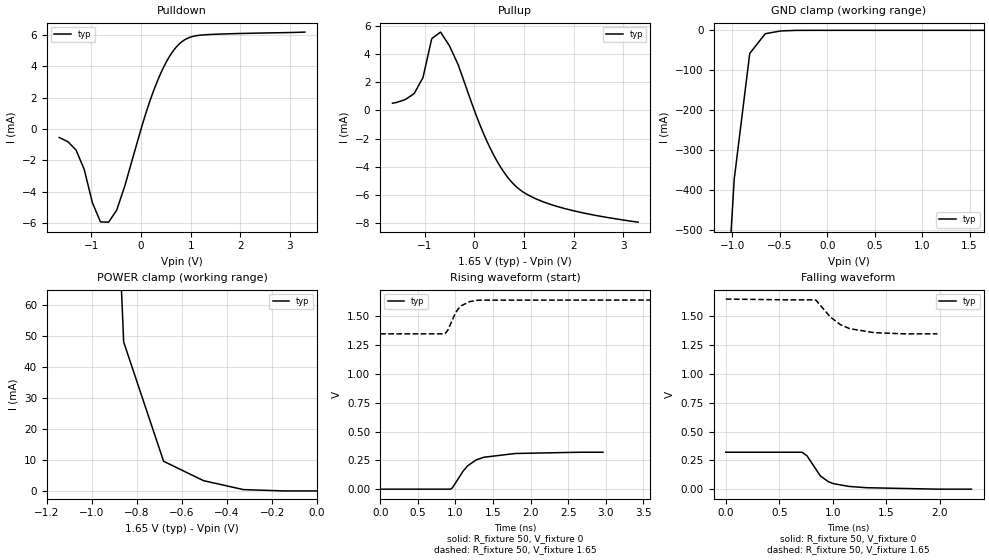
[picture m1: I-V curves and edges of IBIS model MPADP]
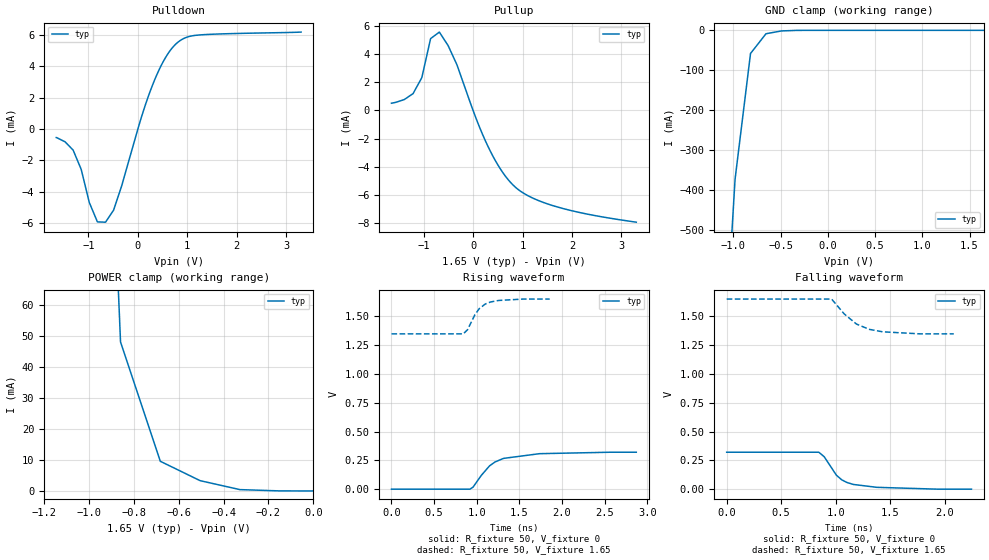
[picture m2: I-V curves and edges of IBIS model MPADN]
| Created by SiliconSmart 2008.10 (Production)
| There are several IBIS sections which it is inappropriate for this tool to
| automatically fill in - copyrights and packaging details are two examples.
| We are making it easy for you to add these things by providing commented-out
| section headers and brief descriptions of each such section.  Of course, the
| IBIS standard is the ultimate section description; these are merely summaries.
[IBIS Ver]   4.1
[File Name]   ss_1p08_1p65_125c.ibs
[File Rev]   1.0
[Date]   December 18 11:21:58
[Source]   From SiliconSmart 2008.10 (Production)
|[Notes]   Use this section for any special notes related to the file.
|   (fill in and uncomment to use this section)
|[Disclaimer]   Legal disclaimer section.
|   (fill in and uncomment to use this section)
|[Copyright]   Copyright 1995, XYZ Corp., All Rights Reserved
|   (fill in and uncomment to use this section)
[Component]   pdqs_ddr2_cl_driver_6p9ma
[Manufacturer]   Unknown
[Package]
| Variable   typ   min   max
R_pkg   18   NA   NA
L_pkg   1n   NA   NA
C_pkg   15f   NA   NA
[Pin]   signal_name   model_name   R_pin   L_pin   C_pin
1   PADP   MPADP   NA   NA   NA
2   PADN   MPADN   NA   NA   NA
3   DVSS   GND   NA   NA   NA
4   DVDD   POWER   NA   NA   NA
|[Package Model]   Package model name.  40-char limit.
|   (fill in and uncomment to use this section)
[Pin Mapping]  pulldown_ref   pullup_ref   gnd_clamp_ref  power_clamp_ref
1   DVSS   DVDD   DVSS   DVDD
2   DVSS   DVDD   DVSS   DVDD
3   DVSS   NC   NC   NC
4   NC   DVDD   NC   NC
[Diff Pin]  inv_pin  vdiff  tdelay_typ tdelay_min tdelay_max
1   2   NA   -36.38p   NA   NA
| Models and submodels in the file (2): MPADP (I/O), MPADN (I/O)
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|PADP pin
[Model]   MPADP
Model_type I/O
Polarity Non-Inverting
Vinl = 0.8
Vinh = 2.0
Vmeas = 0.9
| Capacitance   typ   min   max
C_comp   6.42p   NA   NA
| Variables   typ   min   max
[Temperature Range]   125   NA   NA
[Voltage Range]   1.65   NA   NA
[Pullup Reference]   1.65   NA   NA
[Pulldown Reference]   0.0   NA   NA
[POWER Clamp Reference]   1.65   NA   NA
[GND Clamp Reference]   0.0   NA   NA
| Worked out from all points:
|   slope of the pulldown table from 0 to 0.247 V, typ, clamps not added: 103 ohm
|   slope of the pullup table from 0 to 0.247 V, typ, clamps not added: 115 ohm
|   GND clamp passes 1 mA (typ) near -0.43 V on its own axis
|   POWER clamp passes 1 mA (typ) near -0.36 V on its own axis
|   falling waveform, R_fixture 50, V_fixture 0: 20-80 % time 178ps typ, NA min, NA max; typ from 0.321 V to 0 V
|   falling waveform, R_fixture 50, V_fixture 1.65: 20-80 % time 230ps typ, NA min, NA max; typ from 1.65 V to 1.35 V
|   rising waveform, R_fixture 50, V_fixture 0: 20-80 % time 277ps typ, NA min, NA max; typ from 0 V to 0.321 V
|   rising waveform, R_fixture 50, V_fixture 1.65: 20-80 % time 156ps typ, NA min, NA max; typ from 1.35 V to 1.65 V
[Pulldown]
| Voltage   I(typ)   I(min)   I(max)
-1.65V    -547uA     NA         NA
-1.309V   -1.35mA    NA         NA
-1.145V   -2.589mA   NA         NA
-981.8mV  -4.706mA   NA         NA
-818.2mV  -5.944mA   NA         NA
-654.5mV  -5.963mA   NA         NA
-490.9mV  -5.192mA   NA         NA
309.4mV   2.913mA    NA         NA
534.4mV   4.436mA    NA         NA
759.4mV   5.412mA    NA         NA
1.209V    6.007mA    NA         NA
3.3V      6.201mA    NA         NA
[GND Clamp]
| Voltage   I(typ)   I(min)   I(max)
-1.65V    -3.783A    NA         NA
-1.145V   -1.023A    NA         NA
-981.8mV  -373.2mA   NA         NA
-818.2mV  -58.01mA   NA         NA
-654.5mV  -8.539mA   NA         NA
-490.9mV  -1.513mA   NA         NA
-327.3mV  -141.6uA   NA         NA
1.65V     207.2nA    NA         NA
[Pullup]
| Voltage   I(typ)   I(min)   I(max)
-1.65V    512.4uA    NA         NA
-1.214V   1.194mA    NA         NA
-1.036V   2.33mA     NA         NA
-859.1mV  5.1mA      NA         NA
-681.8mV  5.564mA    NA         NA
-327.3mV  3.249mA    NA         NA
46.88mV   -441.6uA   NA         NA
300mV     -2.544mA   NA         NA
553.1mV   -4.162mA   NA         NA
806.3mV   -5.29mA    NA         NA
1.65V     -6.801mA   NA         NA
3.3V      -7.938mA   NA         NA
[POWER Clamp]
| Voltage   I(typ)   I(min)   I(max)
-1.65V    3.52A      NA         NA
-1.036V   353.3mA    NA         NA
-859.1mV  48.02mA    NA         NA
-681.8mV  9.556mA    NA         NA
-504.5mV  3.311mA    NA         NA
-327.3mV  425.7uA    NA         NA
0V        0A         NA         NA
[Ramp]
dV/dt_r   0.186742/0.216555n NA   NA
dV/dt_f   0.186741/0.203874n NA   NA
R_load = 50
[Falling Waveform]
R_fixture = 50
V_fixture = 0
| Time   V(typ)   V(min)   V(max)
0s        320.6mV    NA         NA
711ps     320.6mV    NA         NA
757.3ps   290.7mV    NA         NA
883.7ps   114.8mV    NA         NA
957.2ps   64.99mV    NA         NA
1.004ns   48.22mV    NA         NA
1.15ns    23.9mV     NA         NA
1.315ns   12.63mV    NA         NA
1.982ns   44.78uV    NA         NA
2.295ns   44.78uV    NA         NA
[Falling Waveform]
R_fixture = 50
V_fixture = 1.65
| Time   V(typ)   V(min)   V(max)
0s        1.65V      NA         NA
572.1ps   1.643V     NA         NA
815.3ps   1.643V     NA         NA
840.7ps   1.642V     NA         NA
977.2ps   1.493V     NA         NA
1.073ns   1.427V     NA         NA
1.157ns   1.393V     NA         NA
1.382ns   1.359V     NA         NA
1.665ns   1.348V     NA         NA
1.977ns   1.348V     NA         NA
[Rising Waveform]
R_fixture = 50
V_fixture = 0
| Time   V(typ)   V(min)   V(max)
0s        45.5uV     NA         NA
933.2ps   45.5uV     NA         NA
960.6ps   12.32mV    NA         NA
1.102ns   156.3mV    NA         NA
1.162ns   202.5mV    NA         NA
1.274ns   253.1mV    NA         NA
1.377ns   276.8mV    NA         NA
1.797ns   309.7mV    NA         NA
2.65ns    320.6mV    NA         NA
2.962ns   320.6mV    NA         NA
[Rising Waveform]
R_fixture = 50
V_fixture = 1.65
| Time   V(typ)   V(min)   V(max)
0s        1.348V     NA         NA
850.2ps   1.348V     NA         NA
869.7ps   1.355V     NA         NA
897.9ps   1.379V     NA         NA
1.001ns   1.529V     NA         NA
1.033ns   1.562V     NA         NA
1.078ns   1.592V     NA         NA
1.189ns   1.628V     NA         NA
1.305ns   1.641V     NA         NA
31.56ns   1.65V      NA         NA
|PADN pin
[Model]   MPADN
Model_type I/O
Polarity Inverting
Vinl = 0.8
Vinh = 2.0
Vmeas = 0.9
| Capacitance   typ   min   max
C_comp   6.42p   NA   NA
| Variables   typ   min   max
[Temperature Range]   125   NA   NA
[Voltage Range]   1.65   NA   NA
[Pullup Reference]   1.65   NA   NA
[Pulldown Reference]   0.0   NA   NA
[POWER Clamp Reference]   1.65   NA   NA
[GND Clamp Reference]   0.0   NA   NA
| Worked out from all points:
|   slope of the pulldown table from 0 to 0.247 V, typ, clamps not added: 103 ohm
|   slope of the pullup table from 0 to 0.247 V, typ, clamps not added: 115 ohm
|   GND clamp passes 1 mA (typ) near -0.43 V on its own axis
|   POWER clamp passes 1 mA (typ) near -0.36 V on its own axis
|   falling waveform, R_fixture 50, V_fixture 0: 20-80 % time 178ps typ, NA min, NA max; typ from 0.321 V to 0 V
|   falling waveform, R_fixture 50, V_fixture 1.65: 20-80 % time 237ps typ, NA min, NA max; typ from 1.65 V to 1.35 V
|   rising waveform, R_fixture 50, V_fixture 0: 20-80 % time 279ps typ, NA min, NA max; typ from 0 V to 0.321 V
|   rising waveform, R_fixture 50, V_fixture 1.65: 20-80 % time 161ps typ, NA min, NA max; typ from 1.35 V to 1.65 V
[Pulldown]
| Voltage   I(typ)   I(min)   I(max)
-1.65V    -547uA     NA         NA
-1.309V   -1.35mA    NA         NA
-1.145V   -2.589mA   NA         NA
-981.8mV  -4.706mA   NA         NA
-818.2mV  -5.944mA   NA         NA
-654.5mV  -5.963mA   NA         NA
-490.9mV  -5.192mA   NA         NA
309.4mV   2.913mA    NA         NA
534.4mV   4.436mA    NA         NA
759.4mV   5.412mA    NA         NA
1.209V    6.007mA    NA         NA
3.3V      6.201mA    NA         NA
[GND Clamp]
| Voltage   I(typ)   I(min)   I(max)
-1.65V    -3.783A    NA         NA
-1.145V   -1.023A    NA         NA
-981.8mV  -373.2mA   NA         NA
-818.2mV  -58.01mA   NA         NA
-654.5mV  -8.539mA   NA         NA
-490.9mV  -1.513mA   NA         NA
-327.3mV  -141.6uA   NA         NA
1.65V     207.2nA    NA         NA
[Pullup]
| Voltage   I(typ)   I(min)   I(max)
-1.65V    512.4uA    NA         NA
-1.214V   1.194mA    NA         NA
-1.036V   2.33mA     NA         NA
-859.1mV  5.1mA      NA         NA
-681.8mV  5.564mA    NA         NA
-327.3mV  3.249mA    NA         NA
46.88mV   -441.6uA   NA         NA
300mV     -2.544mA   NA         NA
553.1mV   -4.162mA   NA         NA
806.3mV   -5.29mA    NA         NA
1.65V     -6.801mA   NA         NA
3.3V      -7.938mA   NA         NA
[POWER Clamp]
| Voltage   I(typ)   I(min)   I(max)
-1.65V    3.52A      NA         NA
-1.036V   353.3mA    NA         NA
-859.1mV  48.02mA    NA         NA
-681.8mV  9.556mA    NA         NA
-504.5mV  3.311mA    NA         NA
-327.3mV  425.7uA    NA         NA
0V        0A         NA         NA
[Ramp]
dV/dt_r   0.186742/0.220127n NA   NA
dV/dt_f   0.18674/0.207349n NA   NA
R_load = 50
[Falling Waveform]
R_fixture = 50
V_fixture = 0
| Time   V(typ)   V(min)   V(max)
0s        320.6mV    NA         NA
844.6ps   320.6mV    NA         NA
894ps     281.4mV    NA         NA
1.006ns   120.7mV    NA         NA
1.055ns   81.18mV    NA         NA
1.102ns   58.01mV    NA         NA
1.162ns   40.87mV    NA         NA
1.377ns   15.98mV    NA         NA
1.932ns   45.5uV     NA         NA
2.244ns   45.5uV     NA         NA
[Falling Waveform]
R_fixture = 50
V_fixture = 1.65
| Time   V(typ)   V(min)   V(max)
0s        1.65V      NA         NA
961.7ps   1.65V      NA         NA
967.1ps   1.644V     NA         NA
1.078ns   1.521V     NA         NA
1.189ns   1.434V     NA         NA
1.305ns   1.388V     NA         NA
1.429ns   1.366V     NA         NA
1.653ns   1.354V     NA         NA
1.769ns   1.348V     NA         NA
2.082ns   1.348V     NA         NA
[Rising Waveform]
R_fixture = 50
V_fixture = 0
| Time   V(typ)   V(min)   V(max)
0s        45.51uV    NA         NA
920.7ps   45.51uV    NA         NA
957.2ps   18.21mV    NA         NA
1.053ns   119.7mV    NA         NA
1.15ns    202.1mV    NA         NA
1.214ns   236mV      NA         NA
1.315ns   267.3mV    NA         NA
1.736ns   308mV      NA         NA
2.559ns   320.6mV    NA         NA
2.871ns   320.6mV    NA         NA
[Rising Waveform]
R_fixture = 50
V_fixture = 1.65
| Time   V(typ)   V(min)   V(max)
0s        1.348V     NA         NA
842.6ps   1.348V     NA         NA
892.1ps   1.384V     NA         NA
978.1ps   1.514V     NA         NA
1.028ns   1.566V     NA         NA
1.099ns   1.606V     NA         NA
1.158ns   1.624V     NA         NA
1.255ns   1.638V     NA         NA
1.543ns   1.65V      NA         NA
1.856ns   1.65V      NA         NA
